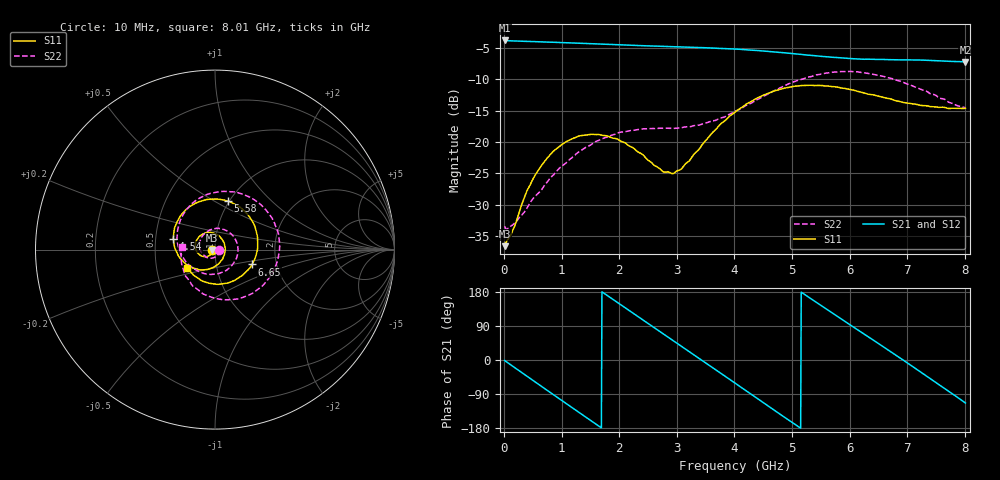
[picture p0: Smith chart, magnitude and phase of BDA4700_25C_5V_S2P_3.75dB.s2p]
!Agilent Technologies,E5071B,MY42404982,A.09.10
!Date: Mon Oct 20 13:27:46 2025
!Data & Calibration Information:
!Freq	S11:SOLT2(ON)	S21:SOLT2(ON)	S12:SOLT2(ON)	S22:SOLT2(ON)
# Hz S RI R 50
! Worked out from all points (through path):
!   801 points, 10 MHz to 8.01 GHz, reference 50 ohm
!   highest |S21| = -3.86 dB at 10 MHz (marker M1); lowest = -7.3 dB at 8.01 GHz (marker M2)
!   group delay of S21, straight-line fit = 288 ps
!   lowest |S11| = -36.5 dB at 10 MHz (marker M3), VSWR 1.03, Z = 48.5 - j0.147 ohm
!   |S11| at or under -10 dB: start of sweep to end of sweep
!   |S22| runs from -33.8 to -8.8 dB; largest |S21 - S12| = 0.0046
!   S11 on the Smith chart (normalised r, x): 10 MHz: 0.97, -0.00; 4.54 GHz: 0.62, +0.08; 5.58 GHz: 0.99, +0.58; 6.65 GHz: 1.49, -0.26; 8.01 GHz: 0.72, -0.15
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1e7  -0.0148 -0.00151  0.6408 -0.014  0.641 -0.0141  0.0213 -0.00181
3.3e8  -0.0231 -0.025  0.5138 -0.3675  0.5134 -0.368  0.0199 -0.0181
7.2e8  -0.0598 -0.0394  0.1406 -0.6068  0.1405 -0.6069  -0.00727 -0.0457
1.02e9  -0.0942 -0.0212  -0.1966 -0.5837  -0.1971 -0.584  -0.0509 -0.0407
1.35e9  -0.1101 0.024  -0.4882 -0.3625  -0.4888 -0.3631  -0.0857 0.0112
1.92e9  -0.0539 0.0924  -0.5463 0.2333  -0.5464 0.2337  -0.013 0.1145
2.32e9  0.0114 0.0828  -0.2492 0.5285  -0.2489 0.5286  0.0894 0.0882
2.68e9  0.0509 0.0361  0.1215 0.5642  0.1214 0.5641  0.1282 -0.00554
2.95e9  0.0548 -0.014  0.369 0.4364  0.3689 0.4359  0.1026 -0.0768
3.36e9  0.0132 -0.084  0.559 0.0701  0.5598 0.0699  0.00744 -0.1357
3.66e9  -0.0531 -0.1119  0.5078 -0.2277  0.5073 -0.229  -0.0757 -0.1272
4.01e9  -0.1472 -0.0903  0.2667 -0.4785  0.2667 -0.4782  -0.1596 -0.0703
4.54e9  -0.232 0.0598  -0.2358 -0.4708  -0.2358 -0.4715  -0.2078 0.1102
4.95e9  -0.1757 0.2076  -0.4741 -0.1789  -0.4746 -0.1801  -0.1157 0.2667
5.35e9  -0.028 0.2805  -0.4561 0.1706  -0.4567 0.1698  0.0828 0.3227
5.58e9  0.0711 0.2694  -0.3434 0.3298  -0.3436 0.3305  0.2059 0.2856
6.09e9  0.2229 0.1276  0.0425 0.4563  0.0435 0.4575  0.3588 0.0457
6.65e9  0.2065 -0.0829  0.3978 0.2135  0.3985 0.2128  0.2374 -0.2225
6.68e9  0.2012 -0.0924  0.4081 0.1919  0.4089 0.1914  0.2246 -0.232
7.23e9  0.048 -0.1896  0.382 -0.2333  0.3821 -0.2344  -0.0308 -0.2613
7.62e9  -0.0698 -0.1759  0.1339 -0.4197  0.1331 -0.4204  -0.1638 -0.1478
8.01e9  -0.1541 -0.1033  -0.1713 -0.3974  -0.1713 -0.3981  -0.1866 0.0151
